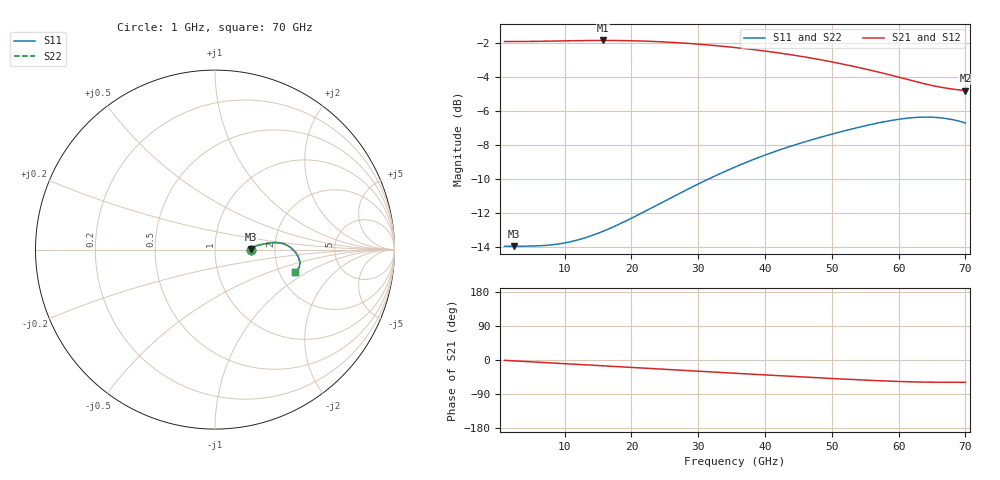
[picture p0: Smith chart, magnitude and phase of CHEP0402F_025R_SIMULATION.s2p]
! Touchstone file exported from HFSS 2026.1.0
!  File:  S:/COMPOSANTS_3D_CRYPTES/CHEP0402F/2026R1/PCB_&_COMP/PCB_V1.1.003_CHEP0402F_V1.aedt
!  $RV = 25ohm
# GHz S MA R 50.000000
! Terminal data exported
! Port[1] = LINE_T1
! Port[2] = LINE_T2
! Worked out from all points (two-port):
!   401 points, 1 GHz to 70 GHz, reference 50 ohm
!   highest |S21| = -1.88 dB at 15.66 GHz (marker M1); lowest = -4.8 dB at 70 GHz (marker M2)
!   |S21| within 3 dB of the highest: start of sweep to end of sweep
!   lowest |S11| = -14.0 dB at 2.38 GHz (marker M3), VSWR 1.50, Z = 75 + j0.0956 ohm
!   |S11| at or under -10 dB: start of sweep to 31.66 GHz
!   |S22| runs from -14.0 to -6.4 dB; largest |S21 - S12| = 6.9e-14
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1  0.2002 0.0  0.7998 -0.9  0.7998 -0.9  0.2002 0.0
2.38  0.2001 0.2  0.8001 -2.3  0.8001 -2.3  0.2001 0.2
8.0725  0.2019 1.6  0.8023 -7.8  0.8023 -7.8  0.202 1.6
10.315  0.2051 2.4  0.8038 -10.0  0.8038 -10.0  0.2052 2.4
12.5575  0.2103 3.3  0.805 -12.2  0.805 -12.2  0.2104 3.3
15.6625  0.221 4.4  0.8058 -15.3  0.8058 -15.3  0.2211 4.4
19.8025  0.2407 5.6  0.8043 -19.5  0.8043 -19.5  0.2409 5.6
24.115  0.2661 6.4  0.7991 -23.9  0.7991 -23.9  0.2663 6.4
29.8075  0.3036 6.8  0.7865 -29.5  0.7865 -29.5  0.3038 6.9
35.5  0.342 6.5  0.7681 -35.0  0.7681 -35.0  0.3422 6.5
38.605  0.3621 5.9  0.7559 -38.0  0.7559 -38.0  0.3623 5.9
41.5375  0.3802 5.0  0.743 -40.9  0.743 -40.9  0.3804 5.1
44.2975  0.3963 3.9  0.7294 -43.5  0.7294 -43.5  0.3965 4.0
47.0575  0.4116 2.5  0.7144 -46.1  0.7144 -46.1  0.4119 2.6
49.99  0.4272 0.8  0.697 -48.8  0.697 -48.8  0.4274 0.9
52.9225  0.4421 -1.1  0.6782 -51.4  0.6782 -51.4  0.4424 -1.0
55.855  0.4561 -3.3  0.6584 -53.7  0.6584 -53.7  0.4564 -3.2
58.615  0.4677 -5.5  0.6388 -55.8  0.6388 -55.8  0.468 -5.4
61.72  0.477 -8.3  0.6158 -57.6  0.6158 -57.6  0.4773 -8.2
64.48  0.4796 -10.9  0.5971 -58.5  0.5971 -58.5  0.4799 -10.8
67.0675  0.4751 -13.2  0.5836 -58.9  0.5836 -58.9  0.4755 -13.2
70  0.4607 -15.6  0.5738 -58.7  0.5738 -58.7  0.4611 -15.5
